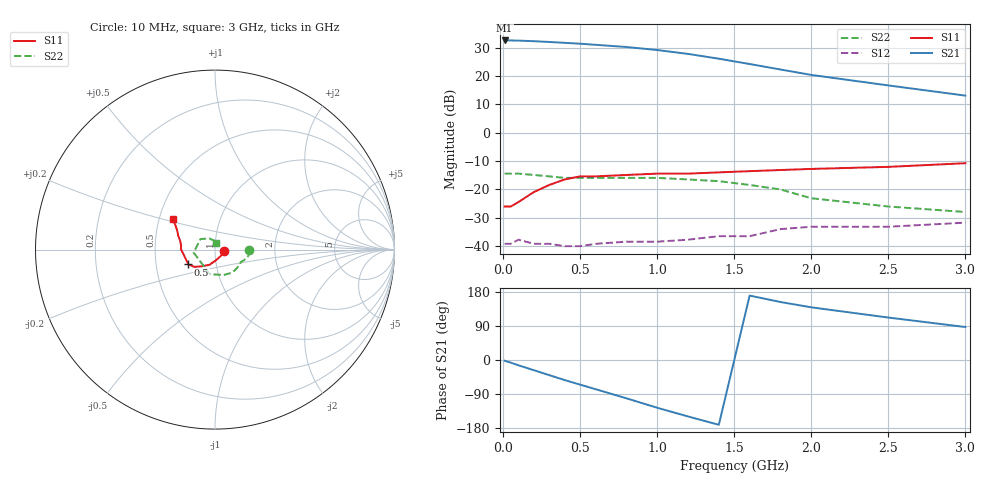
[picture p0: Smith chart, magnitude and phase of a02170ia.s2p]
!  INA-02170  S PARAMETERS
!  Id = 35 mA  LAST UPDATED 07-22-92
# ghz s ma r 50
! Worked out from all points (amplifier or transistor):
!   17 points, 10 MHz to 3 GHz, reference 50 ohm
!   highest |S21| = 32.5 dB at 10 MHz (marker M1)
!   |S21| within 3 dB of that: start of sweep to 930 MHz
!   unconditionally stable (mu >= 1): start of sweep to end of sweep
!   at 100 MHz: K = 1.15, MAG = 32.7 dB, |S12| = -37.7 dB
!   at 800 MHz: K = 1.43, MAG = 30.4 dB, |S12| = -38.4 dB
!   at 3 GHz: K = 3.96, MAG = 13.5 dB, |S12| = -31.7 dB
!   lowest NFmin = 1.60 dB at 100 MHz
!   S11 on the Smith chart (normalised r, x): 10 MHz: 1.10, -0.02; 500 MHz: 0.73, -0.12; 3 GHz: 0.59, +0.22
0.01  0.05 -8.0  42.32 -2.0  0.011 14.0  0.19 -1.0
0.05  0.05 -31.0  42.32 -7.0  0.011 14.0  0.19 -5.0
0.1  0.06 -85.0  42.05 -14.0  0.013 10.0  0.19 -10.0
0.2  0.09 -110.0  41.06 -27.0  0.011 5.0  0.18 -16.0
0.3  0.12 -129.0  39.82 -40.0  0.011 1.0  0.17 -21.0
0.4  0.15 -140.0  38.43 -53.0  0.01 19.0  0.16 -25.0
0.5  0.17 -151.0  37.08 -65.0  0.01 8.0  0.16 -27.0
0.6  0.17 -159.0  35.49 -77.0  0.011 23.0  0.16 -30.0
0.8  0.18 -174.0  32.45 -101.0  0.012 23.0  0.16 -40.0
1  0.19 179.0  28.7 -126.0  0.012 17.0  0.16 -53.0
1.2  0.19 173.0  24.51 -149.0  0.013 27.0  0.15 -71.0
1.4  0.2 166.0  20.18 -171.0  0.015 35.0  0.14 -102.0
1.6  0.21 162.0  16.26 170.0  0.015 34.0  0.12 -172.0
1.8  0.22 159.0  13.02 153.0  0.02 46.0  0.1 144.0
2  0.23 155.0  10.45 139.0  0.022 37.0  0.07 117.0
2.5  0.25 150.0  6.82 112.0  0.022 32.0  0.05 95.0
3  0.29 144.0  4.51 87.0  0.026 32.0  0.04 78.0
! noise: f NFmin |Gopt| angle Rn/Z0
0.1  1.6  0.23  2  0.3
0.5  1.7  0.21  10  0.29
1  1.9  0.14  19  0.3
2  2.8  0.05  -137  0.32
